TYPE dut_Interlock :
STRUCT
	Alarm1		: BOOL;	// N2-8 pressure low
	Alarm2		: BOOL;	// N2-1 pressure low or high
	Alarm3		: BOOL;	// NH3-1 pressure low or high
	Alarm4		: BOOL;	// NH3-2 pressure low or high
	Alarm5		: BOOL;	// SiH4 pressure low or high
	Alarm6		: BOOL;	// N2-2 pressure low or high
	Alarm7		: BOOL;	// NF3 pressure low or high
	Alarm8		: BOOL;	// 20%F2/N2 pressure low or high
	Alarm9		: BOOL;	// N2-9 pressure low or high
	Alarm10		: BOOL;	// N2-10 pressure low or high
	Alarm11		: BOOL;	// N2-11 pressure low or high
	Alarm12		: BOOL;	// N2-13 pressure low or high
	Alarm13		: BOOL;	// LSC tank over pressure
	Alarm14		: BOOL;	// TI tank over pressure
	Alarm15		: BOOL;	// NH3-1 tank over pressure
	Alarm16		: BOOL;	// Vacuum pressure low
	Alarm17		: BOOL;	// air/N2-1 pressure low
	Alarm18		: BOOL;	// N2-4 pressure low
	Alarm19		: BOOL;	// N2-5 pressure low
	Alarm20		: BOOL;	// N2-6 pressure low
	Alarm21		: BOOL;	// NH3-2 tank over pressure
	Alarm22		: BOOL;	// gas box lower and upper exhaust pressure low
	Alarm23		: BOOL;	// Scavenger exhaust pressure low
	Alarm24		: BOOL;	// Heater exhaust pressure low
	Alarm25		: BOOL;	// RHC pressure low
	Alarm26		: BOOL;	// Z purge in LSC-1 pressure
	Alarm27		: BOOL;	// Gas box lower an upper exhaust pressure low
	Alarm28		: BOOL;	// Abnormal diaphragm sensor reading value
	Alarm29		: BOOL;	// spare
	Alarm30		: BOOL;	// Abnormal furnace port cap seal level
	Alarm31		: BOOL;	// Heater exceeds the upper limit
	Alarm32		: BOOL;	// Heater room temperature high
	Alarm33		: BOOL;	// spare
	Alarm34		: BOOL;	// Heater transformer temperature high
	Alarm35		: BOOL;	// spare
	Alarm36		: BOOL;   // AC100V transformer temperature high
	Alarm37		: BOOL;   // spare
	Alarm38		: BOOL;	// spare
	Alarm39		: BOOL;	// N2 does not flow in each foup
	Alarm40		: BOOL;	// Exhaust pressure high
	Alarm41		: BOOL;	// Power down detected
	Alarm42		: BOOL;	// Front door kept open
	Alarm43		: BOOL;	// Transfer room door kept open
	Alarm44		: BOOL;	// Heater room door kept open
	Alarm45		: BOOL;	// Heater power down
	Alarm46		: BOOL;	// spare
	Alarm47		: BOOL;	// Pump down
	Alarm48		: BOOL;	// Pump alarm
	Alarm49		: BOOL;	// Pump warning
	Alarm50		: BOOL;	// spare
	Alarm51		: BOOL;	// NH3 leak detection
	Alarm52		: BOOL;	// SiH4 leak detection
	Alarm53		: BOOL;	// HCL leak detection
	Alarm54		: BOOL;	// Diaphgram sensor-VG11 negative value
	Alarm55		: BOOL;	// Diaphgram sensor-VG13 negative value
	Alarm56		: BOOL;	// Diaphgram sensor-VG14 negative value
	Alarm57		: BOOL;	// APC alarm
	Alarm58		: BOOL;	// Too high furnace pressure
	Alarm59		: BOOL;	// Main cooling water flow low
	Alarm60		: BOOL;	// Cooling water flow low
	Alarm61		: BOOL;	// NF3 gas leak detection
	Alarm62		: BOOL;	// 20%F2/N2 leak detection
	Alarm63		: BOOL;	// scrubber NG DEPO
	Alarm64		: BOOL;	// scrubber NG CLN
	Alarm65		: BOOL;	// FFU stop
	Alarm66		: BOOL;	// SPARE
	Alarm67		: BOOL;	// Loading area differential pressure abnormal
	Alarm68		: BOOL;	// Clean unit temperature high
	Alarm69		: BOOL;	// Differential pressure NG-DG1
	Alarm70		: BOOL; // RHC flow low
	Alarm71		: BOOL;	// RHC damper abnormal position
	Alarm72		: BOOL;	// Blower overload
	Alarm73		: BOOL;	// RHC cooling water bypass line flow low/damper position abnormal in energy-saving mode
	Alarm74		: BOOL;	// Cooling water pressure low
	Alarm75		: BOOL;	// TI tank refll incorrect
	Alarm76		: BOOL;	// Abnormal float sw position in TI tank
	Alarm77		: BOOL;	// N2-7 pressure low or high
	Alarm78		: BOOL;	// N2-70 pressure low or high
	Alarm79		: BOOL;	// Vent exhaust pressure high
	Alarm80		: BOOL;	// Gas box door kept open
	Alarm81		: BOOL;	// Magnetic leak
	Alarm82		: BOOL;	// Heater room leak
	Alarm83		: BOOL;	// Loading area leak
	Alarm84		: BOOL;	// Exhaust box main leak
	Alarm85		: BOOL;	// SPARE
	Alarm86		: BOOL;	// RHC leak
	Alarm87		: BOOL;	// Exhaust box sup leak
	Alarm88		: BOOL;	// O2 analyzer fault
	Alarm89		: BOOL;	// Heater contactor tripped
	Alarm90		: BOOL;	// AC100V transformer contactor tripped
	Alarm91		: BOOL;	// gas box door kept open
	Alarm92		: BOOL;	// spare
	Alarm93		: BOOL;	// spare
	Alarm94		: BOOL;	// failure of exhaust pressure sensor
	Alarm95		: BOOL;	// Transfer room EMS
	Alarm96		: BOOL;	// Furnace pressure is below ATM pressure
	Alarm97		: BOOL; // Front body exhaust pressure low
	Alarm98		: BOOL;	// Gage valve position error
	Alarm99		: BOOL;	// LSC heater temperature abnormal
	Alarm100	: BOOL;	// Gas line heater temperature abnormal
	Alarm101	: BOOL;	// Exhaust line heater temperature abnormal
	Alarm102	: BOOL;	// VG11/13/14 heater temperature abnormal
	Alarm103	: BOOL;	// Seal cap heater temperature high
	Alarm104	: BOOL;	// spare
	Alarm105	: BOOL;	// Furnace & exhaust line heater temperature beyond a preset value
	Alarm106	: BOOL;	// Intake damper position abnormal
	Alarm107	: BOOL;	// ATM damper position abnormal
	Alarm108	: BOOL;	// Cycle damper position abnormal
	Alarm109	: BOOL;	// LSC tank level HH
	Alarm110	: BOOL;	// LSC tank level H
	Alarm111	: BOOL;	// LSC tank level M
	Alarm112	: BOOL;	// LSC tank level L
	Alarm113	: BOOL;	// LSC leak
	Alarm114	: BOOL;	// spare
	Alarm115	: BOOL;	// sspare
	Alarm116	: BOOL;	// HPM interlock
	Alarm117	: BOOL;	// Scrubber alarm
	Alarm118	: BOOL;	// Foreline heater alarm
	Alarm119	: BOOL;	// Scrubber warning
	Alarm120	: BOOL;	// spare
	Alarm121	: BOOL;	// Customer's auto refill alarm
	Alarm122	: BOOL;	// Customer's auto refill warning
	Alarm123	: BOOL;	// Customer's auto refill bulk empty(not ready)
	Alarm124	: BOOL;	// Gas detector trouble
	Alarm125	: BOOL;	// External EMO in
	Alarm126	: BOOL;	// spare
	Alarm127	: BOOL;	// spare
	Alarm128	: BOOL;	// spare
	Alarm129	: BOOL;	// spare
	Alarm130	: BOOL;	// spare
	Alarm131	: BOOL;	// spare
	Alarm132	: BOOL;	// spare
	Alarm133	: BOOL;	// spare
	Alarm134	: BOOL;	// spare
	Alarm135	: BOOL;	// spare
	Alarm136	: BOOL;	// spare
	Alarm137	: BOOL;	// spare
	Alarm138	: BOOL;	// spare
	Alarm139	: BOOL;	// spare
	Alarm140	: BOOL;	// spare
	Alarm141	: BOOL;	// spare
	Alarm142	: BOOL;	// spare
	Alarm143	: BOOL;	// spare
	Alarm144	: BOOL;	// spare
	Alarm145	: BOOL;	// spare
	Alarm146	: BOOL;	// spare
	Alarm147	: BOOL;	// spare
	Alarm148	: BOOL;	// spare
	Alarm149	: BOOL;	// spare
	Alarm150	: BOOL;	// spare
	
END_STRUCT
END_TYPE
